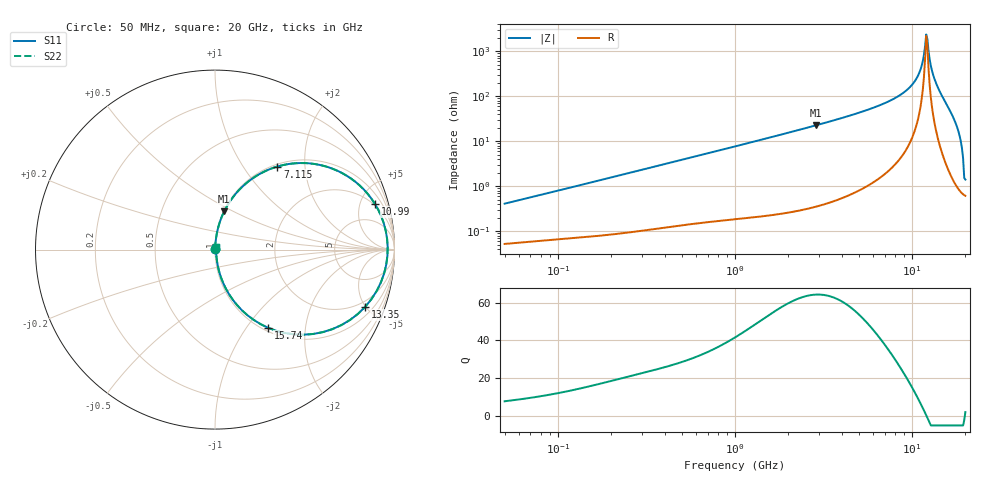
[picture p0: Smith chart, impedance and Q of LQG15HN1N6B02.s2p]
!Murata Part Number: LQG15HN1N6B02
!These Parameters are Measured in Series Mode Connection
!  o--[Z]--o
!Port1  Port2
!  o-------o
!Freq. Start=50[MHz] Stop=20[GHz], 401[Steps]
# Hz S RI R 50
!Freq.(Hz) S11(Real) S11(Imag) S21(Real) S21(Imag) S12(Real) S12(Imag) S22(Real) S22(Imag)
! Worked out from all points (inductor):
!   401 points, 50 MHz to 20 GHz, reference 50 ohm
!   read as one part in series: L = 1.29 nH near 51.52 MHz
!   highest Q = 64.2 at 2.853 GHz (marker M1), where L = 1.26 nH
!   self-resonance near 12.02 GHz
!   S11 on the Smith chart (normalised r, x): 50 MHz: 1.00, +0.01; 7.115 GHz: 1.04, +1.45; 10.99 GHz: 1.84, +6.64; 13.35 GHz: 1.54, -4.97; 15.74 GHz: 1.05, -1.28; 20 GHz: 1.01, +0.03
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5e7  0.000541 0.00407  0.9995 -0.00407  0.9995 -0.00407  0.000541 0.00407
1.364002e8  0.000849 0.0108  0.9992 -0.0108  0.9992 -0.0108  0.000849 0.0108
3.721004e8  0.00199 0.0289  0.998 -0.0289  0.998 -0.0289  0.00199 0.0289
1e9  0.00769 0.0761  0.9923 -0.0761  0.9923 -0.0761  0.00769 0.0761
2.728004e9  0.047 0.204  0.953 -0.204  0.953 -0.204  0.047 0.204
2.853386e9  0.0513 0.213  0.9487 -0.213  0.9487 -0.213  0.0513 0.213
4.89267e9  0.1535 0.3514  0.8465 -0.3514  0.8465 -0.3514  0.1535 0.3514
7.114996e9  0.3472 0.4627  0.6528 -0.4627  0.6528 -0.4627  0.3472 0.4627
7.442007e9  0.3845 0.4721  0.6155 -0.4721  0.6155 -0.4721  0.3845 0.4721
9.600142e9  0.6885 0.4362  0.3115 -0.4362  0.3115 -0.4362  0.6885 0.4362
1.098561e10  0.8911 0.2547  0.1089 -0.2547  0.1089 -0.2547  0.8911 0.2547
1.183995e10  0.9587 0.061  0.0413 -0.061  0.0413 -0.061  0.9587 0.061
1.201863e10  0.962 0.0147  0.038 -0.0147  0.038 -0.0147  0.962 0.0147
1.238412e10  0.9543 -0.0827  0.0457 0.0827  0.0457 0.0827  0.9543 -0.0827
1.276073e10  0.9246 -0.1819  0.0754 0.1819  0.0754 0.1819  0.9246 -0.1819
1.334722e10  0.8366 -0.3191  0.1634 0.3191  0.1634 0.3191  0.8366 -0.3191
1.438523e10  0.6 -0.46  0.4 0.46  0.4 0.46  0.6 -0.46
1.573793e10  0.2972 -0.4361  0.7028 0.4361  0.7028 0.4361  0.2972 -0.4361
1.721783e10  0.0997 -0.2802  0.9003 0.2802  0.9003 0.2802  0.0997 -0.2802
1.828096e10  0.0342 -0.1575  0.9658 0.1575  0.9658 0.1575  0.0342 -0.1575
1.88369e10  0.0171 -0.0979  0.9829 0.0979  0.9829 0.0979  0.0171 -0.0979
2e10  0.00627 0.0125  0.9937 -0.0125  0.9937 -0.0125  0.00627 0.0125
